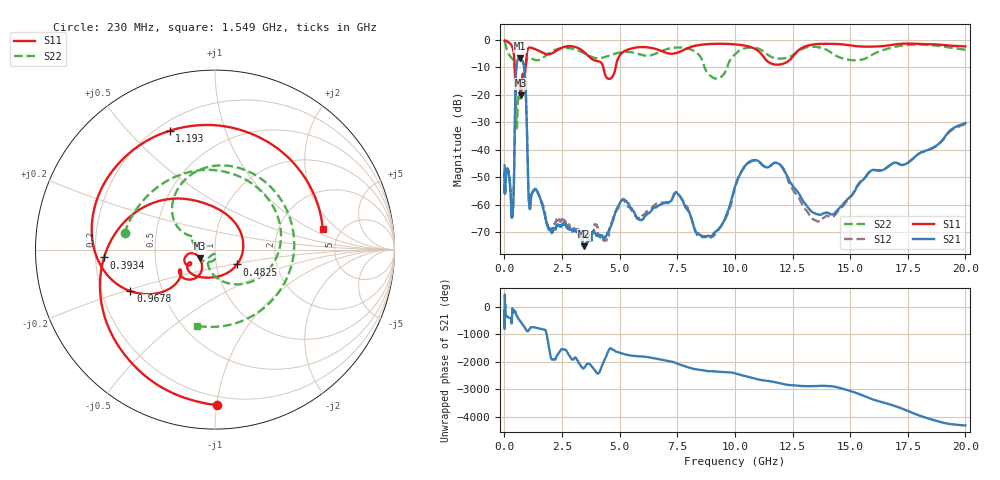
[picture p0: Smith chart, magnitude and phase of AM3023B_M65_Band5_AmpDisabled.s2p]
!Agilent Technologies,E8364B,MY43040894,A.07.50.67
!Agilent E8364B: A.07.50.67
!Date: Tuesday, October 27, 2020 10:49:27
!Correction: S11(Full 2 Port(1,2))
!S21(Full 2 Port(1,2))
!S12(Full 2 Port(1,2))
!S22(Full 2 Port(1,2))
!S2P File: Measurements: S11, S21, S12, S22:Log Frequency Sweep
# Hz S  dB  R 50
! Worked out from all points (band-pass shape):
!   3201 points, 10 MHz to 20 GHz, reference 50 ohm
!   highest |S21| = -6.75 dB at 684.2 MHz (marker M1); lowest = -75.1 dB at 3.441 GHz (marker M2)
!   |S21| within 3 dB of the highest: 520.2 MHz to 852.1 MHz (331.9 MHz wide, 48.4 % of centre)
!   lowest |S11| = -20.2 dB at 702.3 MHz (marker M3), VSWR 1.22, Z = 42 - j4.17 ohm
!   |S11| at or under -10 dB: 444.9 MHz to 916 MHz (471.2 MHz wide, 69.2 % of centre); 4.292 GHz to 4.828 GHz (535.8 MHz wide, 11.7 % of centre)
!   |S22| runs from -32.2 to -0.7 dB; largest |S21 - S12| = 0.0077
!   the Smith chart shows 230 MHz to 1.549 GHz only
!   S11 on the Smith chart (normalised r, x): 230 MHz: 0.14, -1.00; 393.4 MHz: 0.23, -0.03; 482.5 MHz: 1.26, -0.21; 967.8 MHz: 0.33, -0.21; 1.193 GHz: 0.25, +0.66; 1.549 GHz: 3.62, +1.33
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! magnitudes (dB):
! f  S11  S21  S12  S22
! 10 MHz  -0.3  -45.7  -51.4  -0.7
! 35.55 MHz  -0.4  -53.3  -52.9  -1.2
! 126.1 MHz  -0.7  -47.0  -47.2  -4.1
! 230 MHz  -1.2  -51.1  -51.2  -5.8
! 393.4 MHz  -4.2  -57.9  -58.3  -7.4
! 447.2 MHz  -10.6  -34.5  -34.4  -9.1
! 482.5 MHz  -16.6  -16.7  -16.8  -15.1
! 535.7 MHz  -15.0  -8.7  -8.7  -32.2
! 684.2 MHz  -19.5  -6.7  -6.8  -21.4
! 702.3 MHz  -20.2  -6.8  -6.8  -21.3
! 967.8 MHz  -5.6  -29.1  -29.2  -7.4
! 1.072 GHz  -2.9  -59.7  -59.3  -6.5
! 1.193 GHz  -3.0  -56.0  -55.9  -7.0
! 1.549 GHz  -4.3  -57.5  -57.8  -7.2
! 1.59 GHz  -4.4  -58.6  -58.7  -7.0
! 3.441 GHz  -4.4  -75.1  -69.9  -4.9
! 5.639 GHz  -3.0  -62.9  -63.4  -4.8
! 7.534 GHz  -4.7  -56.2  -56.0  -2.8
! 8.897 GHz  -1.6  -71.4  -72.2  -12.9
! 10.86 GHz  -3.3  -43.7  -43.9  -2.9
! 13.87 GHz  -1.5  -63.1  -64.7  -3.3
! 20 GHz  -2.4  -30.3  -30.6  -3.7
